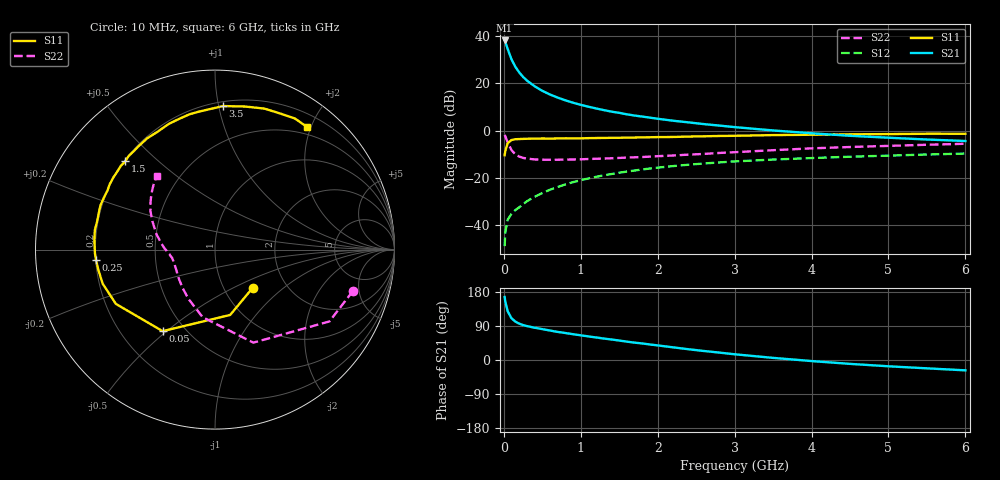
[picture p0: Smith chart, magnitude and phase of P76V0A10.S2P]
! SIEMENS Small Signal Semiconductors
! BFP196
! Si NPN RF Bipolar Junction Transistor in SOT143
! VCE = 6 V  IC = 100 mA
! Common Emitter S-Parameters:  May  1996
# GHz  S  MA  R  50
!  f  S11  S21  S12  S22
! GHz  MAG  ANG  MAG  ANG  MAG  ANG  MAG  ANG
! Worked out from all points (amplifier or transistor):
!   36 points, 10 MHz to 6 GHz, reference 50 ohm
!   highest |S21| = 38.3 dB at 10 MHz (marker M1)
!   |S21| within 3 dB of that: start of sweep to 43.45 MHz
!   unconditionally stable (mu >= 1): 370.6 MHz to 4.565 GHz
!   at 250 MHz: K = 0.92, MSG = 27.0 dB, |S12| = -31.3 dB
!   at 1.4 GHz: K = 1.09, MAG = 11.4 dB, |S12| = -18.5 dB
!   at 6 GHz: K = 0.98, MSG = 2.7 dB, |S12| = -9.8 dB
!   S11 on the Smith chart (normalised r, x): 10 MHz: 1.37, -0.63; 50 MHz: 0.38, -0.48; 250 MHz: 0.20, -0.04; 1.5 GHz: 0.20, +0.39; 3.5 GHz: 0.23, +1.03; 6 GHz: 0.38, +1.94
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0.01  0.2991 -45.0  82.03 166.3  0.0035 76.9  0.8024 -16.7
0.02  0.3737 -76.9  75.14 153.4  0.0071 69.4  0.7528 -32.1
0.05  0.54 -122.7  54.04 128.6  0.0128 54.7  0.5607 -67.6
0.1  0.6298 -151.3  32.42 110.0  0.0171 49.3  0.3831 -100.3
0.15  0.6541 -163.2  22.55 101.3  0.0205 52.8  0.3119 -118.3
0.2  0.6598 -170.3  17.21 95.9  0.0234 55.4  0.2799 -130.1
0.25  0.6656 -175.1  13.78 92.2  0.0273 58.3  0.2625 -138.6
0.3  0.6694 -178.4  11.55 89.5  0.0315 60.7  0.2542 -144.2
0.4  0.6745 175.2  8.732 85.2  0.0392 63.1  0.2434 -152.6
0.5  0.6782 170.8  6.983 81.5  0.0471 64.5  0.2404 -157.9
0.6  0.6753 166.3  5.828 77.7  0.0554 65.0  0.2396 -161.4
0.7  0.6794 162.2  5.013 74.1  0.0633 65.0  0.2402 -164.2
0.9  0.6835 155.2  3.899 68.1  0.0803 63.4  0.2427 -168.4
1.1  0.6902 148.3  3.209 62.2  0.0961 61.4  0.2485 -171.1
1.5  0.7016 135.5  2.378 51.3  0.1273 56.0  0.2622 -176.0
1.7  0.7112 129.4  2.083 45.8  0.1418 53.0  0.2705 -178.8
2.2  0.7306 115.9  1.618 33.4  0.1759 45.4  0.295 174.9
2.8  0.7671 100.7  1.277 19.6  0.2103 36.4  0.3344 165.9
3.5  0.801 86.8  1.005 5.6  0.242 26.2  0.3826 155.7
4.5  0.8324 70.7  0.774 -10.2  0.2781 14.3  0.4473 143.4
5.5  0.8555 58.6  0.645 -22.0  0.3098 3.5  0.4993 133.2
6  0.8541 53.2  0.6 -27.3  0.3246 -2.2  0.5241 128.4
